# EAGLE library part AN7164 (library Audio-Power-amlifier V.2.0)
The AN7164 is an integrated circuit designed for 30 W (VCC = 21 V, 8 W) output power amplifier. High power output (BTL 30 W), low distortion and low noise are realized. High reliability is obtained due to various kinds of protectors built in. Furthermore, on-off of output is possible from standby terminal.
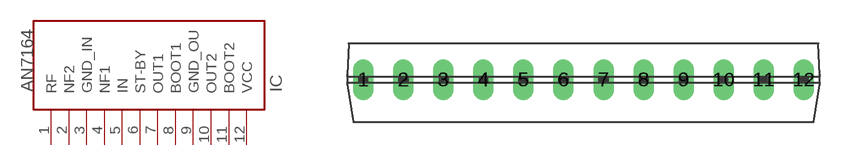
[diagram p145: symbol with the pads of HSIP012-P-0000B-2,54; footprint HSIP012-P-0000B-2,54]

Designator prefix IC

## AN7164  [HSIP012-P-0000B-2,54]
1  RF
2  NF2
3  GND_IN  pwr
4  NF1  in
5  IN  in
6  ST-BY  in
7  OUT1  out
8  BOOT1
9  GND_OU  pwr
10  OUT2  out
11  BOOT2
12  VCC  pwr

## Footprint HSIP012-P-0000B-2,54 (pad centres in mm)
drill 0.8 long: 1 -13.97,0; 2 -11.43,0; 3 -8.89,0; 4 -6.35,0; 5 -3.81,0; 6 -1.27,0; 7 1.27,0; 8 3.81,0; 9 6.35,0; 10 8.89,0; 11 11.43,0; 12 13.97,0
